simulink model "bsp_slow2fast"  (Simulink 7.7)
settings: Solver=FixedStepDiscrete  StartTime=0.0  StopTime=20.0  RelTol=1e-3

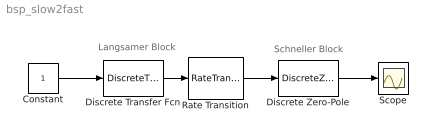
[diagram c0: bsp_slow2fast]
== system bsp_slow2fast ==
  note: Langsamer Block
  note: Schneller Block
  Constant : Constant
  Discrete Transfer Fcn : DiscreteTransferFcn  SampleTime=2
  Discrete Zero-Pole : DiscreteZeroPole  Poles=[0 0.5]  Gain=1
  Rate Transition : RateTransition
  Scope : Scope
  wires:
  Constant/1 -> Discrete Transfer Fcn/1
  Discrete Zero-Pole/1 -> Scope/1
  Discrete Transfer Fcn/1 -> Rate Transition/1
  Rate Transition/1 -> Discrete Zero-Pole/1
